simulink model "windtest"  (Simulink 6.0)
settings: Solver=ode5  SolverMode=SingleTasking  StartTime=0.0  StopTime=15  FixedStep=0.01  RelTol=1e-3  AbsTol=1e-6
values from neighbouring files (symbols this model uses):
  A = [data(3:end-1);data(2:end-2);data(1:end-3)]'    [arfftcomp.m]    (also in arfftcomp2.m = [A,tA(:)]; p192.m)
  B = [data(4:end)']    [arfftcomp.m]    (also in arfftcomp2.m = tB(:); p192.m)
undefined symbols (not defined in the file or in its folder): C, Dd

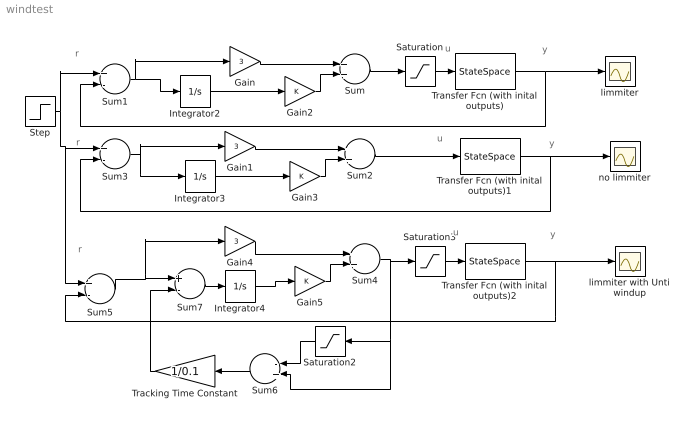
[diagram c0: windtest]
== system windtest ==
  note: r
  note: r
  note: r
  note: u
  note: u
  note: u
  note: y
  note: y
  note: y
  Gain : Gain  Gain=3
  Gain1 : Gain  Gain=3
  Gain2 : Gain
  Gain3 : Gain
  Gain4 : Gain  Gain=3
  Gain5 : Gain
  Integrator2 : Integrator  UpperSaturationLimit=1  LowerSaturationLimit=-1
  Integrator3 : Integrator  UpperSaturationLimit=1  LowerSaturationLimit=-1
  Integrator4 : Integrator  UpperSaturationLimit=1  LowerSaturationLimit=-1
  Saturation : Saturate  UpperLimit=1  LowerLimit=-1
  Saturation2 : Saturate  Orientation=left  UpperLimit=1  LowerLimit=-1
  Saturation3 : Saturate  UpperLimit=1  LowerLimit=-1
  Step : Step  After=0.7
  Sum : Sum
  Sum{1,3,5,7} (4 alike) : Sum  Inputs=+-
  Sum2 : Sum
  Sum4 : Sum
  Sum6 : Sum  Orientation=left  Inputs=-+
  Tracking Time Constant : Gain  Orientation=left  Gain=1/0.1
  Transfer Fcn (with inital outputs) : StateSpace  A=A  B=B  C=C  D=Dd  X0=X0  mask(Transfer Function with Initial Outputs){N=[1], D=[1  -1], Y0=0, U0=0}
      mask prompts: N "Numerator:"; D "Denominator:"; Y0 "Initial Output:"; U0 "Initial Input:"
      mask help: Vector expressions for numerator, and denominator. Coefficients are in descending powers of s.
      mask init:
      | [A,B,C,Dd]=tf2ss(N,D);if (isempty(Y0));[m,n]=size(A);X0=zeros(1,m); end; if (isempty(U0));[m,p]=size(B);U0=zeros(1,p);end;X0=getxo(A,B,C,Dd,U0,Y0,0);
  Transfer Fcn (with inital outputs)1 : StateSpace  A=A  B=B  C=C  D=Dd  X0=X0  mask(Transfer Function with Initial Outputs){N=[1], D=[1  -1], Y0=0, U0=0}
      mask prompts: N "Numerator:"; D "Denominator:"; Y0 "Initial Output:"; U0 "Initial Input:"
      mask help: Vector expressions for numerator, and denominator. Coefficients are in descending powers of s.
      mask init:
      | [A,B,C,Dd]=tf2ss(N,D);if (isempty(Y0));[m,n]=size(A);X0=zeros(1,m); end; if (isempty(U0));[m,p]=size(B);U0=zeros(1,p);end;X0=getxo(A,B,C,Dd,U0,Y0,0);
  Transfer Fcn (with inital outputs)2 : StateSpace  A=A  B=B  C=C  D=Dd  X0=X0  mask(Transfer Function with Initial Outputs){N=[1], D=[1  -1], Y0=0, U0=0}
      mask prompts: N "Numerator:"; D "Denominator:"; Y0 "Initial Output:"; U0 "Initial Input:"
      mask help: Vector expressions for numerator, and denominator. Coefficients are in descending powers of s.
      mask init:
      | [A,B,C,Dd]=tf2ss(N,D);if (isempty(Y0));[m,n]=size(A);X0=zeros(1,m); end; if (isempty(U0));[m,p]=size(B);U0=zeros(1,p);end;X0=getxo(A,B,C,Dd,U0,Y0,0);
  limmiter : Scope
  limmiter with Unti windup : Scope
  no limmiter : Scope
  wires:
  Gain/1 -> Sum/1
  Saturation/1 -> Transfer Fcn (with inital outputs)/1
  Gain2/1 -> Sum/2
  Sum/1 -> Saturation/1
  Integrator2/1 -> Gain2/1
  Sum1/1 -> Gain/1, Integrator2/1
  Transfer Fcn (with inital outputs)/1 -> limmiter/1, Sum1/2
  Gain1/1 -> Sum2/1
  Sum2/1 -> Transfer Fcn (with inital outputs)1/1
  Gain3/1 -> Sum2/2
  Integrator3/1 -> Gain3/1
  Sum3/1 -> Gain1/1, Integrator3/1
  Transfer Fcn (with inital outputs)1/1 -> no limmiter/1, Sum3/2
  Step/1 -> Sum1/1, Sum3/1, Sum5/1
  Gain4/1 -> Sum4/1
  Transfer Fcn (with inital outputs)2/1 -> limmiter with Unti windup/1, Sum5/2
  Saturation2/1 -> Sum6/1
  Saturation3/1 -> Transfer Fcn (with inital outputs)2/1
  Sum4/1 -> Sum6/2, Saturation2/1, Saturation3/1
  Sum7/1 -> Integrator4/1
  Integrator4/1 -> Gain5/1
  Gain5/1 -> Sum4/2
  Sum5/1 -> Gain4/1, Sum7/1
  Tracking Time Constant/1 -> Sum7/2
  Sum6/1 -> Tracking Time Constant/1
